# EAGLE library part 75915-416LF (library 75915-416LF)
Dubox, Board To Board Connector, Receptacle, Vertical, Through Hole, Single Row, Top Entry, 16 Positions, 2.54mm (0.100in) Pitch Source: Datasheet
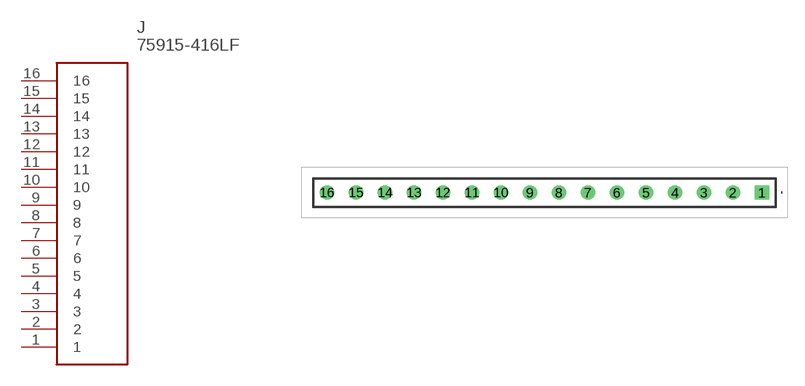
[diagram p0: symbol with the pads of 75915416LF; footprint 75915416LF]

Designator prefix J

## 75915-416LF (Description: Dubox, Board To Board Connector, Receptacle, Vertical, Through Hole, Single Row, Top Entry, 16 Positions, 2.54mm (0.100in) Pitch; Height: 8.8mm; Manufacturer_Name: Amphenol; Manufacturer_Part_Number: 75915-416LF; Mouser_Part_Number: 649-75915-416LF; Mouser_Price-Stock: https://www.mouser.co.uk/ProductDetail/Amphenol-FCI/75915-416LF?qs=eir4yccFG7SFJX2y%252B9zxjQ%3D%3D)  [75915416LF]
1  1
2  2
3  3
4  4
5  5
6  6
7  7
8  8
9  9
10  10
11  11
12  12
13  13
14  14
15  15
16  16

## Footprint 75915416LF (pad centres in mm)
75915-416LF-2
drill 0.75 pad 1.2 square: 1 0,0
drill 0.75 pad 1.2: 2 -2.54,0; 3 -5.08,0; 4 -7.62,0; 5 -10.16,0; 6 -12.7,0; 7 -15.24,0; 8 -17.78,0; 9 -20.32,0; 10 -22.86,0; 11 -25.4,0; 12 -27.94,0; 13 -30.48,0; 14 -33.02,0; 15 -35.56,0; 16 -38.1,0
